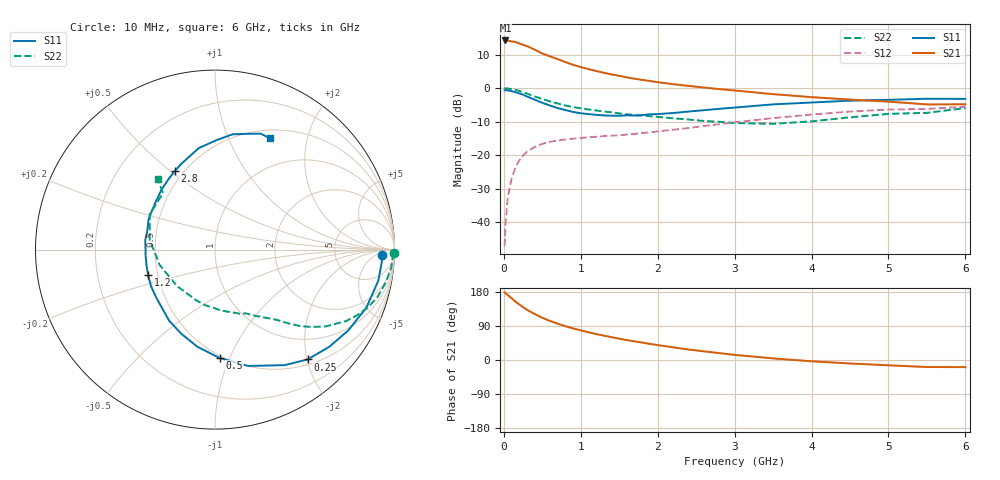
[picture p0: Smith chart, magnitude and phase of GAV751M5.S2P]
! Infineon Technologies  Discrete & RF Semiconductors
! BF775
! Si NPN RF Bipolar Junction Transistor in SOT23
! VCE = 0.75 V  IC = 1.5 mA
! Common Emitter S-Parameters:  May  1996
# GHz  S  MA  R  50
!  f  S11  S21  S12  S22
! GHz  MAG  ANG  MAG  ANG  MAG  ANG  MAG  ANG
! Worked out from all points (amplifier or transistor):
!   36 points, 10 MHz to 6 GHz, reference 50 ohm
!   highest |S21| = 14.2 dB at 20 MHz (marker M1)
!   |S21| within 3 dB of that: start of sweep to 423.2 MHz
!   unconditionally stable (mu >= 1): 1.174 GHz to end of sweep
!   at 250 MHz: K = 0.26, MSG = 16.5 dB, |S12| = -20.1 dB
!   at 1.4 GHz: K = 1.12, MAG = 7.0 dB, |S12| = -14.2 dB
!   at 6 GHz: K = 1.08, MAG = -1.4 dB, |S12| = -5.5 dB
!   S11 on the Smith chart (normalised r, x): 10 MHz: 22, -11; 250 MHz: 0.59, -2.01; 500 MHz: 0.48, -0.92; 1.2 GHz: 0.44, -0.15; 2.8 GHz: 0.45, +0.52; 6 GHz: 0.60, +1.43
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0.01  0.93 -2.0  5.036 178.7  0.0044 88.6  0.9965 -1.1
0.02  0.9317 -4.4  5.14 176.5  0.0091 86.3  0.991 -2.2
0.05  0.9264 -10.7  5.123 171.4  0.023 82.9  0.9873 -5.8
0.1  0.9032 -21.0  4.972 163.2  0.0448 77.4  0.9683 -11.0
0.15  0.8685 -31.2  4.892 154.0  0.0653 70.8  0.9421 -16.5
0.25  0.8004 -49.9  4.429 139.3  0.0989 60.5  0.8708 -25.0
0.3  0.7511 -59.0  4.237 132.4  0.1126 56.4  0.8303 -28.7
0.4  0.674 -74.1  3.753 121.6  0.1325 49.1  0.7513 -34.7
0.5  0.6047 -87.5  3.285 111.4  0.1478 44.0  0.6882 -38.8
0.6  0.5505 -100.2  2.978 103.1  0.1585 39.7  0.6359 -42.0
0.7  0.5044 -112.1  2.706 95.7  0.1657 36.8  0.5898 -44.6
0.8  0.471 -122.9  2.445 89.2  0.1713 34.8  0.5511 -46.8
0.9  0.4411 -131.6  2.229 83.3  0.1764 33.4  0.5212 -48.7
1.1  0.4104 -150.3  1.922 73.2  0.185 31.4  0.481 -52.5
1.2  0.3996 -159.0  1.8 68.5  0.1884 30.7  0.4645 -54.4
1.6  0.3925 172.1  1.445 52.5  0.203 31.5  0.4082 -62.0
2.2  0.4253 140.6  1.146 33.4  0.2396 33.5  0.3549 -77.6
2.8  0.4911 117.3  0.967 18.2  0.2895 32.5  0.3148 -99.9
3.5  0.5726 99.1  0.813 4.2  0.3571 27.5  0.2935 -136.3
4.5  0.6499 81.3  0.675 -9.2  0.4464 15.9  0.3669 171.8
5.5  0.6945 68.5  0.572 -18.5  0.4892 1.8  0.4281 132.6
6  0.6909 63.7  0.573 -18.8  0.529 -2.1  0.5051 129.1
